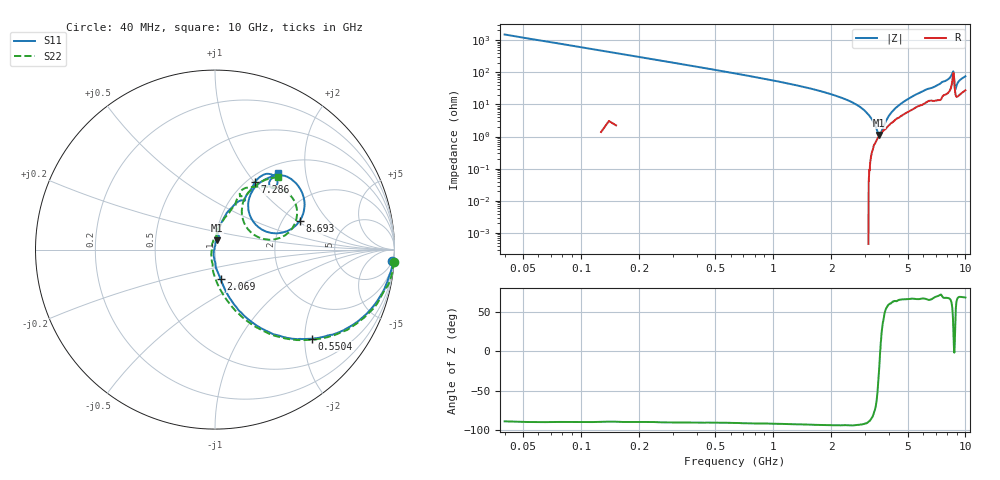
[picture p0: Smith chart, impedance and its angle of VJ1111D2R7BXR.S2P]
! VJ1111D2R7BXR
! DATE 03/04/2022  13:11
! CAPACITORS MOUNTED IN SERIES ON 25 MIL THICK MICROSTRIP SUBSTRATE
# GHz  S  MA  R  50.00
!  FREQ  S11M  S11A  S21M  S21A  S12M  S12A  S22M  S22A
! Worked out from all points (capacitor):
!   801 points, 40 MHz to 10 GHz, reference 50 ohm
!   read as one part in series: C = 2.64 pF near 89.8 MHz
!   lowest |Z| = 1.12 ohm at 3.563 GHz (marker M1)
!   series resonance near 3.602 GHz, so ESL is about 740 pH
!   S11 on the Smith chart (normalised r, x): 40 MHz: 5, -30; 550.5 MHz: 1.01, -2.18; 2.069 GHz: 1.01, -0.34; 7.286 GHz: 1.09, +1.01; 8.693 GHz: 2.47, +1.04; 10 GHz: 1.15, +1.42
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0.04  0.99 -3.7  0.06626 85.4  0.06611 85.6  1.001 -4.0
0.22675  0.9338 -20.2  0.3542 69.7  0.3542 70.3  0.9408 -20.5
0.55045  0.7349 -42.5  0.6903 48.2  0.6932 48.4  0.7344 -43.2
1.02355  0.476 -61.7  0.8969 30.0  0.9002 29.8  0.4695 -63.4
1.7083  0.2475 -74.9  0.9803 17.0  0.9865 16.9  0.2424 -80.7
2.06935  0.1685 -79.2  0.992 12.9  0.9964 12.8  0.164 -89.0
2.79145  0.04958 -96.0  0.9883 7.6  0.9933 7.5  0.05055 -114.0
2.9533  0.02325 -108.9  0.9869 6.9  0.9915 6.6  0.03074 -132.1
3.1027  0.003588 155.9  0.9874 6.0  0.9932 5.8  0.01751 -167.0
3.23965  0.01884 92.1  0.9846 5.2  0.9896 5.0  0.02072 144.6
3.36415  0.03253 87.5  0.9803 4.5  0.9859 4.3  0.02915 122.8
3.56335  0.05334 77.3  0.9796 3.4  0.9855 3.2  0.04628 100.1
3.775  0.07743 72.3  0.9795 2.5  0.9844 2.3  0.07056 88.4
5.02  0.1889 73.8  0.9087 -3.9  0.914 -4.2  0.1635 75.2
6.6883  0.3246 59.1  0.8179 -10.9  0.8225 -11.2  0.2989 66.5
7.2859  0.4375 59.3  0.7952 -14.5  0.8003 -14.8  0.3332 63.6
8.34415  0.5449 49.2  0.6607 -21.3  0.6655 -21.5  0.4718 47.3
8.5558  0.5837 37.2  0.5497 -20.4  0.5526 -20.7  0.5158 36.6
8.69275  0.4971 18.5  0.5022 0.1  0.5048 -0.5  0.4477 15.5
8.8297  0.2641 36.5  0.7595 -0.1  0.7637 -0.4  0.2159 37.4
9.16585  0.4368 56.6  0.7512 -15.9  0.7551 -16.3  0.4066 58.4
10  0.5539 50.7  0.6517 -21.9  0.6563 -22.4  0.5325 49.0
